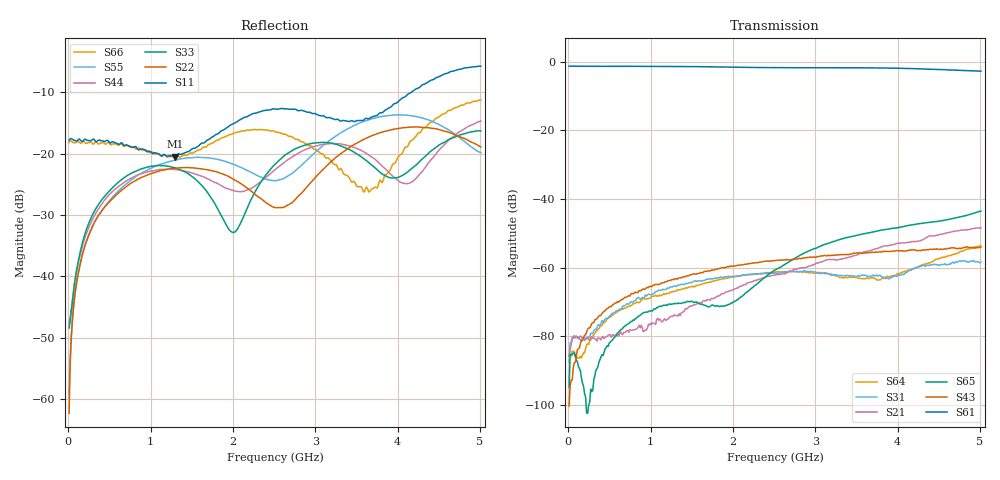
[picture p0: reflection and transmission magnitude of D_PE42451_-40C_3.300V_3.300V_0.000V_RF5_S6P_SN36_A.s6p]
! Device ID: PE42451
! Serial: 36
! Insertion: A
! Temp: -40C
! VDD: 3.300
! Control_Hi: 100.000
! Control_Lo: 0.000
! Logic State: RF5
! Port 1: RFC
! Port 2: RF1
! Port 3: RF2
! Port 4: RF3
! Port 5: RF4
! Port 6: RF5
! V1 = 3.30
! V2 = 0.00
! V3 = 3.30
! V4 = 0.00
! IDD: 1.606380e-05
#  Hz  S  RI  R  50
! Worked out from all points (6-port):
!   401 points, 10 MHz to 5.01 GHz, reference 50 ohm
!   strongest paths, dB at 10 MHz, 1.26 GHz, 2.51 GHz, 3.76 GHz, 5.01 GHz:
!     S61: -1.3, -1.4, -1.7, -1.8, -2.7
!     S43: -100.3, -63.4, -57.9, -55.5, -54.0
!     S65: -94.9, -70.6, -60.7, -49.3, -43.5
!     S21: -87.5, -74.2, -62.2, -54.3, -48.4
!     S31: -85.8, -65.7, -61.6, -62.4, -58.4
!     S64: -85.7, -67.1, -61.2, -63.6, -53.6
!   lowest |S11| = -20.5 dB at 1.298 GHz (marker M1), VSWR 1.21, Z = 53.8 - j9.11 ohm
!   |S11| at or under -10 dB: start of sweep to 4.167 GHz
